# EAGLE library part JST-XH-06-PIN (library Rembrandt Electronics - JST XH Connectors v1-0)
JST XH Connector 2 Pin Wire to board connector. Pitch: 2,54 mm, (0.100") Number of pins: 6 Created by Rembrandt Electronics www.rembrandtelectronics.com
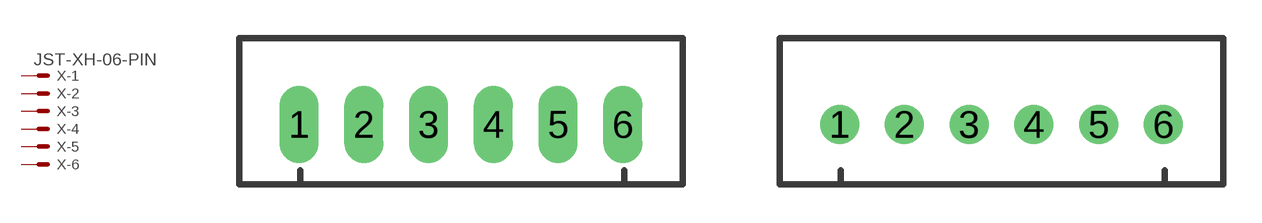
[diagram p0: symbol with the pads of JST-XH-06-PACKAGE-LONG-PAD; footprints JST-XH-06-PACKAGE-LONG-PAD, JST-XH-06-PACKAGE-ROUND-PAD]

Designator prefix X; gates -1=MV -2=M -3=M -4=M -5=M -6=M

## JST-XH-06-PIN-LONG-PAD  [JST-XH-06-PACKAGE-LONG-PAD]
1  -1:S  pas
2  -2:S  pas
3  -3:S  pas
4  -4:S  pas
5  -5:S  pas
6  -6:S  pas

## JST-XH-06-PIN-ROUND-PAD  [JST-XH-06-PACKAGE-ROUND-PAD]
Pads as for JST-XH-06-PACKAGE-LONG-PAD

## Footprint JST-XH-06-PACKAGE-LONG-PAD (pad centres in mm)
JST XH Connector Long Pads (Package) Wire to board connector. Pitch: 2,54 mm, (0.100") Number of pins: 6 Created by Rembrandt Electronics www.rembrandtelectronics.com
drill 1.016 long: 1 -6.35,0; 2 -3.81,0; 3 -1.27,0; 4 1.27,0; 5 3.81,0; 6 6.35,0

## Footprint JST-XH-06-PACKAGE-ROUND-PAD (pad centres in mm)
JST XH Connector Round Pads (Package) Wire to board connector. Pitch: 2,54 mm, (0.100") Number of pins: 6 Created by Rembrandt Electronics www.rembrandtelectronics.com
drill 1.016: 1 -6.35,0; 2 -3.81,0; 3 -1.27,0; 4 1.27,0; 5 3.81,0; 6 6.35,0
